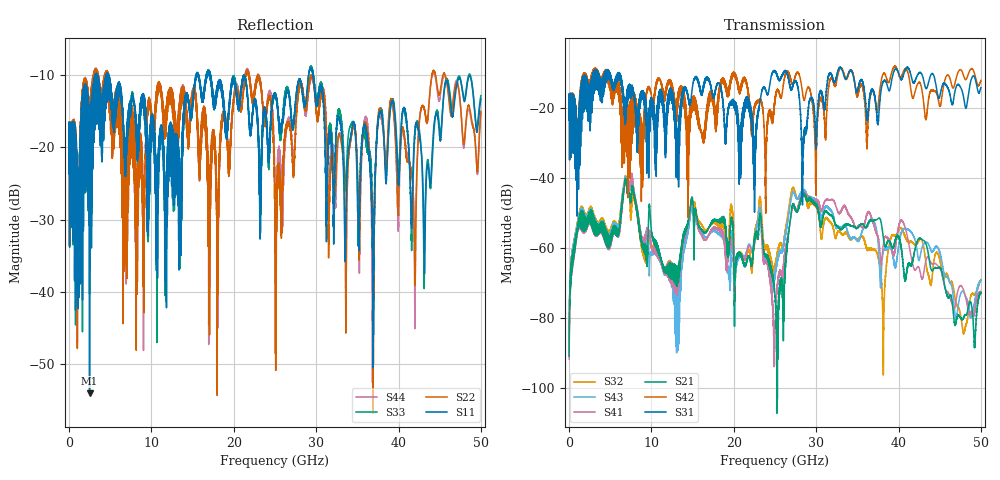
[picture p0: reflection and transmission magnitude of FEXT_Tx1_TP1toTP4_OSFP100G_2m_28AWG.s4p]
! Touchstone data
! Created: 27-Feb-2019 by IdEM 12 (12.1.0)
! COMMENTS
!  Created Wed Feb 27 12:03:36 2019
!  64 Port Network Data from SP1.SP block
!  freq  magS1_1  angS1_1  magS1_2  angS1_2  magS1_3  angS1_3  magS1_4  angS1_4
!  magS1_5  angS1_5  magS1_6  angS1_6  magS1_7  angS1_7  magS1_8  angS1_8
!  magS1_9  angS1_9  magS1_10  angS1_10  magS1_11  angS1_11  magS1_12  angS1_12
!  magS1_13  angS1_13  magS1_14  angS1_14  magS1_15  angS1_15  magS1_16  angS1_16
!  magS1_17  angS1_17  magS1_18  angS1_18  magS1_19  angS1_19  magS1_20  angS1_20
!  magS1_21  angS1_21  magS1_22  angS1_22  magS1_23  angS1_23  magS1_24  angS1_24
!  magS1_25  angS1_25  magS1_26  angS1_26  magS1_27  angS1_27  magS1_28  angS1_28
!  magS1_29  angS1_29  magS1_30  angS1_30  magS1_31  angS1_31  magS1_32  angS1_32
!  magS1_33  angS1_33  magS1_34  angS1_34  magS1_35  angS1_35  magS1_36  angS1_36
!  magS1_37  angS1_37  magS1_38  angS1_38  magS1_39  angS1_39  magS1_40  angS1_40
!  magS1_41  angS1_41  magS1_42  angS1_42  magS1_43  angS1_43  magS1_44  angS1_44
!  magS1_45  angS1_45  magS1_46  angS1_46  magS1_47  angS1_47  magS1_48  angS1_48
!  magS1_49  angS1_49  magS1_50  angS1_50  magS1_51  angS1_51  magS1_52  angS1_52
!  magS1_53  angS1_53  magS1_54  angS1_54  magS1_55  angS1_55  magS1_56  angS1_56
!  magS1_57  angS1_57  magS1_58  angS1_58  magS1_59  angS1_59  magS1_60  angS1_60
!  magS1_61  angS1_61  magS1_62  angS1_62  magS1_63  angS1_63  magS1_64  angS1_64
!  magS2_1  angS2_1  magS2_2  angS2_2  magS2_3  angS2_3  magS2_4  angS2_4
!  magS2_5  angS2_5  magS2_6  angS2_6  magS2_7  angS2_7  magS2_8  angS2_8
!  magS2_9  angS2_9  magS2_10  angS2_10  magS2_11  angS2_11  magS2_12  angS2_12
!  magS2_13  angS2_13  magS2_14  angS2_14  magS2_15  angS2_15  magS2_16  angS2_16
!  magS2_17  angS2_17  magS2_18  angS2_18  magS2_19  angS2_19  magS2_20  angS2_20
!  magS2_21  angS2_21  magS2_22  angS2_22  magS2_23  angS2_23  magS2_24  angS2_24
!  magS2_25  angS2_25  magS2_26  angS2_26  magS2_27  angS2_27  magS2_28  angS2_28
!  magS2_29  angS2_29  magS2_30  angS2_30  magS2_31  angS2_31  magS2_32  angS2_32
!  magS2_33  angS2_33  magS2_34  angS2_34  magS2_35  angS2_35  magS2_36  angS2_36
!  magS2_37  angS2_37  magS2_38  angS2_38  magS2_39  angS2_39  magS2_40  angS2_40
!  magS2_41  angS2_41  magS2_42  angS2_42  magS2_43  angS2_43  magS2_44  angS2_44
!  magS2_45  angS2_45  magS2_46  angS2_46  magS2_47  angS2_47  magS2_48  angS2_48
!  magS2_49  angS2_49  magS2_50  angS2_50  magS2_51  angS2_51  magS2_52  angS2_52
!  magS2_53  angS2_53  magS2_54  angS2_54  magS2_55  angS2_55  magS2_56  angS2_56
!  magS2_57  angS2_57  magS2_58  angS2_58  magS2_59  angS2_59  magS2_60  angS2_60
!  magS2_61  angS2_61  magS2_62  angS2_62  magS2_63  angS2_63  magS2_64  angS2_64
!  magS3_1  angS3_1  magS3_2  angS3_2  magS3_3  angS3_3  magS3_4  angS3_4
!  magS3_5  angS3_5  magS3_6  angS3_6  magS3_7  angS3_7  magS3_8  angS3_8
!  magS3_9  angS3_9  magS3_10  angS3_10  magS3_11  angS3_11  magS3_12  angS3_12
!  magS3_13  angS3_13  magS3_14  angS3_14  magS3_15  angS3_15  magS3_16  angS3_16
!  magS3_17  angS3_17  magS3_18  angS3_18  magS3_19  angS3_19  magS3_20  angS3_20
!  magS3_21  angS3_21  magS3_22  angS3_22  magS3_23  angS3_23  magS3_24  angS3_24
!  magS3_25  angS3_25  magS3_26  angS3_26  magS3_27  angS3_27  magS3_28  angS3_28
!  magS3_29  angS3_29  magS3_30  angS3_30  magS3_31  angS3_31  magS3_32  angS3_32
!  magS3_33  angS3_33  magS3_34  angS3_34  magS3_35  angS3_35  magS3_36  angS3_36
!  magS3_37  angS3_37  magS3_38  angS3_38  magS3_39  angS3_39  magS3_40  angS3_40
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# Hz S MA R 50
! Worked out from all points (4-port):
!   5000 points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, 10 MHz to 50 GHz, reference 50 ohm
!   strongest paths, dB at 10 MHz, 12.51 GHz, 25.01 GHz, 37.51 GHz, 50 GHz:
!     S31: -18.0, -16.4, -9.6, -24.1, -14.3
!     S42: -18.0, -13.2, -17.6, -19.8, -12.3
!     S21: -90.9, -64.6, -74.0, -51.7, -72.9
!     S41: -91.7, -64.4, -82.5, -56.8, -72.6
!     S43: -89.8, -66.2, -67.3, -58.1, -69.2
!     S32: -89.0, -64.8, -65.0, -62.4, -69.0
!   lowest |S11| = -54.1 dB at 2.49 GHz (marker M1), VSWR 1.00, Z = 49.8 + j0.0446 ohm
!   |S11| at or under -10 dB: 4.81 GHz to 15.41 GHz (10.6 GHz wide, 105 % of centre); 17.19 GHz to 29.09 GHz (11.9 GHz wide, 51.4 % of centre); 29.64 GHz to end of sweep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
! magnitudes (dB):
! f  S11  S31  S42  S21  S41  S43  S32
! 10 MHz  -17.7  -18.0  -18.0  -90.9  -91.7  -89.8  -89.0
! 2.49 GHz  -54.1  -22.3  -16.4  -51.7  -52.2  -51.1  -50.6
! 13.08 GHz  -21.8  -27.2  -18.0  -65.8  -65.5  -71.7  -67.9
! 14.88 GHz  -15.0  -16.1  -20.6  -46.1  -47.2  -48.1  -48.0
! 24.93 GHz  -12.9  -9.4  -18.7  -71.7  -93.6  -68.0  -65.4
! 28.46 GHz  -13.3  -30.1  -17.4  -45.1  -44.8  -43.9  -44.6
! 50 GHz  -13.3  -14.3  -12.3  -72.9  -72.6  -69.2  -69.0
